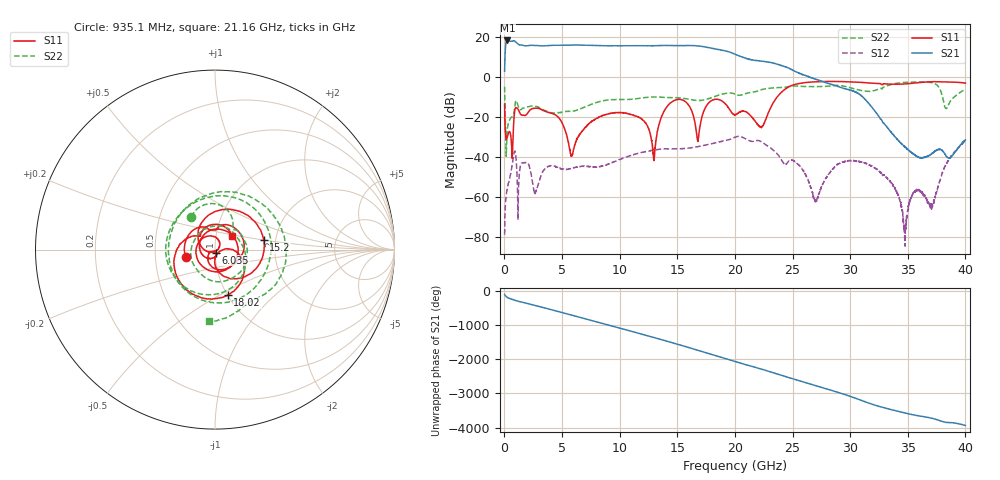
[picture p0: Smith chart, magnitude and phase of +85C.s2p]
#  HZ  S  DB  R  50.00
! Rohde & Schwarz Vector Network Analyzer
! Rohde-Schwarz,ZNB3032-4Port,1351505034101534,4.21
! Created: UTC 6/10/2026, 1:46:18 PM
! freq[Hz]  db:S11  ang:S11  db:S21  ang:S21  db:S12  ang:S12  db:S22  ang:S22
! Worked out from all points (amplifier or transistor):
!   3200 points, 10 MHz to 40 GHz, reference 50 ohm
!   highest |S21| = 18.3 dB at 260 MHz (marker M1)
!   |S21| within 3 dB of that: 91.63 MHz to 17.12 GHz (17.03 GHz wide, 198 % of centre)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
!   unconditionally stable (mu >= 1): start of sweep to end of sweep
!   at 6.673 GHz: K = 13.30, MAG = 16.0 dB, |S12| = -44.7 dB
!   at 20.01 GHz: K = 3.78, MAG = 12.0 dB, |S12| = -30.1 dB
!   at 40 GHz: K = 274.38, MAG = -27.2 dB, |S12| = -31.8 dB
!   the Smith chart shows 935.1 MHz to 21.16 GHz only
!   S11 on the Smith chart (normalised r, x): 935.1 MHz: 0.72, -0.07; 6.035 GHz: 1.01, -0.03; 15.2 GHz: 1.73, +0.20; 18.02 GHz: 1.01, -0.55; 21.16 GHz: 1.20, +0.19
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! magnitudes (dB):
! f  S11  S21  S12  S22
! 10 MHz  -13.5  2.9  -78.8  -4.9
! 260 MHz  -29.5  18.3  -55.1  -25.4
! 935.1 MHz  -15.6  17.7  -37.5  -13.0
! 2.685 GHz  -15.6  15.8  -58.0  -14.7
! 6.035 GHz  -35.4  16.0  -45.3  -17.0
! 6.685 GHz  -27.4  15.9  -44.6  -15.7
! 10.61 GHz  -18.2  15.6  -39.9  -11.2
! 12.95 GHz  -41.2  15.7  -36.5  -10.0
! 13.35 GHz  -25.0  15.7  -36.2  -10.0
! 15.2 GHz  -11.2  15.7  -35.8  -10.4
! 16.77 GHz  -31.9  15.5  -34.8  -11.7
! 18.02 GHz  -11.6  14.3  -33.3  -10.2
! 20.01 GHz  -18.8  11.3  -30.1  -8.5
! 21.16 GHz  -18.2  9.0  -31.6  -8.0
! 26.67 GHz  -2.5  -0.4  -56.9  -4.8
! 29.84 GHz  -2.4  -6.3  -41.7  -5.1
! 33.34 GHz  -3.5  -26.1  -51.2  -4.1
! 34.77 GHz  -3.5  -35.1  -76.6  -2.7
! 35.64 GHz  -3.0  -39.2  -57.4  -2.5
! 37.14 GHz  -2.4  -38.1  -64.9  -2.9
! 38.35 GHz  -2.5  -39.6  -43.3  -15.7
! 40 GHz  -3.0  -31.4  -31.8  -6.0
